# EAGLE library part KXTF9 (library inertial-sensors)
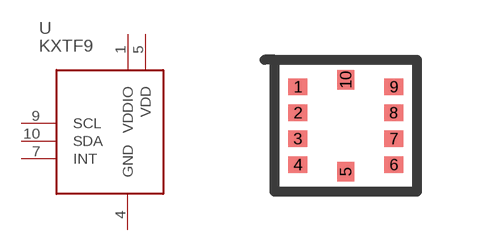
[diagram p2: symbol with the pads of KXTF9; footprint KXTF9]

Designator prefix U

## KXTF9  [KXTF9]
1  VDDIO
4  GND
5  VDD
7  INT
9  SCL
10  SDA

## Footprint KXTF9 (pad centres in mm)
smd 0.48 x 0.42: 1 -1.2,0.975; 2 -1.2,0.325; 3 -1.2,-0.325; 4 -1.2,-0.975; 6 1.2,-0.975; 7 1.2,-0.325; 8 1.2,0.325; 9 1.2,0.975
smd 0.42 x 0.48: 5 0,-1.15; 10 0,1.15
